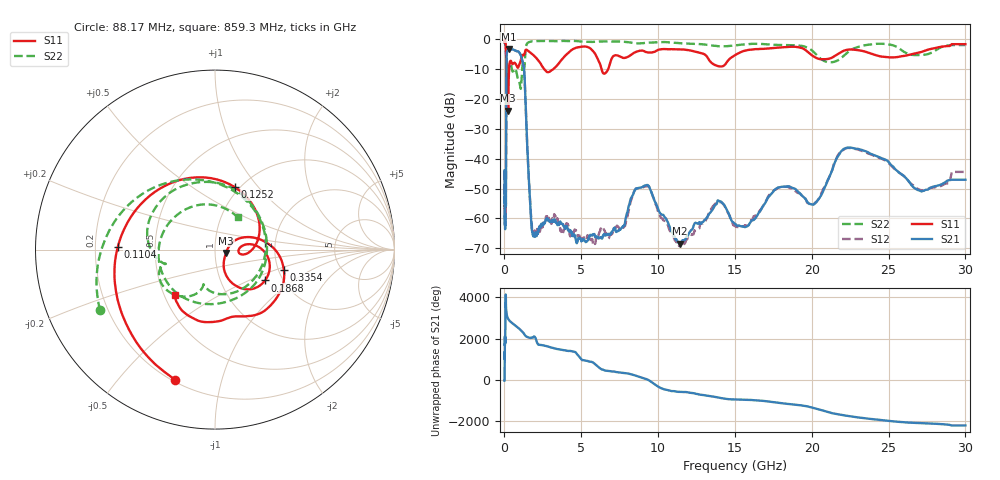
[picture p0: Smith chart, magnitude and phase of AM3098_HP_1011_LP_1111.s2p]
! Date/Time: Thu, Feb 28, 2019 8:43 AM
! Network Analyzer: Agilent Technologies E8364B Rev: A.07.50.67
! Sweep from 0.010 to 30.000 GHz, 1601 Points, Sweep Type: LOG
! Power Supply: 5.022 V, 0.002 A
# Hz S DB R 50
!freq MagS11 AngS11 MagS21 AngS21 MagS12 AngS12 MagS22 AngS22
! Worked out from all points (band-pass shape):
!   1601 points, 10 MHz to 30 GHz, reference 50 ohm
!   highest |S21| = -3.17 dB at 263.8 MHz (marker M1); lowest = -68.5 dB at 11.42 GHz (marker M2)
!   |S21| within 3 dB of the highest: 137.5 MHz to 1.115 GHz (977.2 MHz wide, 156 % of centre)
!   lowest |S11| = -23.9 dB at 242.3 MHz (marker M3), VSWR 1.14, Z = 56.5 - j2.17 ohm
!   |S11| at or under -10 dB: 193.3 MHz to 301.8 MHz (108.6 MHz wide, 43.9 % of centre); 2.6 GHz to 3.17 GHz (570.9 MHz wide, 19.8 % of centre); 6.323 GHz to 6.743 GHz (420.5 MHz wide, 6.44 % of centre)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
!   |S22| runs from -16.5 to -0.5 dB; largest |S21 - S12| = 0.012
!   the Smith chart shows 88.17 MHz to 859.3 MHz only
!   S11 on the Smith chart (normalised r, x): 88.17 MHz: 0.21, -0.72; 110.4 MHz: 0.30, +0.01; 125.2 MHz: 0.95, +0.76; 186.8 MHz: 1.62, -0.62; 335.4 MHz: 2.14, -0.57; 859.3 MHz: 0.57, -0.32
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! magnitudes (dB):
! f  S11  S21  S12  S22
! 10 MHz  -0.3  -43.9  -44.0  -0.6
! 38.04 MHz  -0.4  -58.7  -61.5  -1.0
! 49.1 MHz  -0.7  -51.4  -48.9  -1.3
! 88.17 MHz  -2.4  -53.0  -55.4  -2.8
! 110.4 MHz  -5.3  -32.4  -32.3  -6.7
! 125.2 MHz  -8.8  -12.4  -12.4  -11.1
! 144.7 MHz  -17.5  -5.1  -5.1  -13.8
! 186.8 MHz  -9.7  -3.8  -3.8  -9.0
! 242.3 MHz  -23.9  -3.2  -3.1  -10.9
! 263.8 MHz  -16.4  -3.2  -3.1  -10.4
! 335.4 MHz  -8.0  -3.4  -3.4  -8.0
! 550.5 MHz  -8.2  -3.4  -3.3  -10.7
! 859.3 MHz  -9.5  -4.0  -3.9  -13.1
! 1.263 GHz  -5.3  -9.4  -9.4  -9.9
! 1.758 GHz  -4.7  -62.6  -60.8  -0.6
! 2.084 GHz  -6.3  -65.9  -64.3  -0.5
! 7.926 GHz  -6.1  -59.2  -60.7  -0.8
! 9.21 GHz  -4.2  -48.9  -49.2  -1.1
! 11.42 GHz  -3.3  -68.5  -69.3  -1.2
! 20.1 GHz  -5.6  -55.4  -55.4  -4.1
! 22.67 GHz  -3.4  -36.4  -36.5  -3.2
! 30 GHz  -1.6  -47.0  -44.4  -1.9
